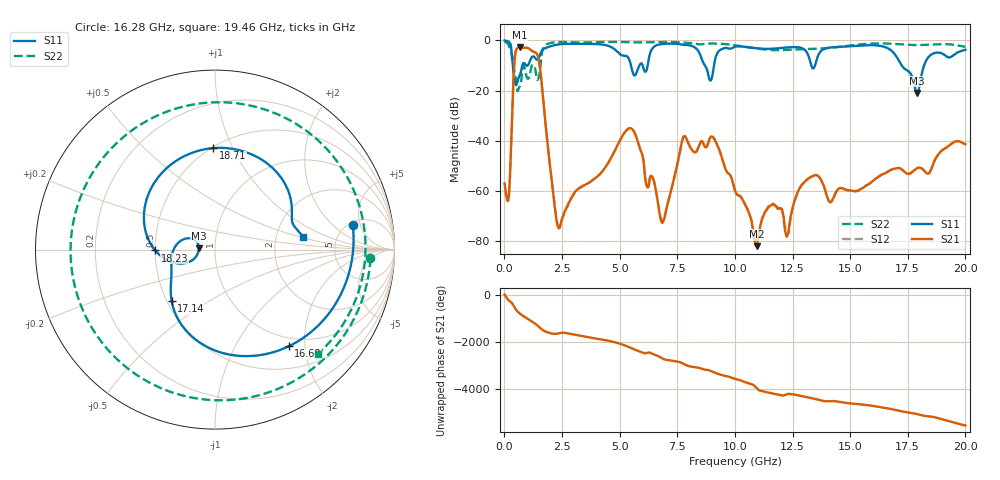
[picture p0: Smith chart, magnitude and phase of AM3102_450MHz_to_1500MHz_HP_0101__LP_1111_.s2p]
!Agilent Technologies,E8364B,MY43040894,A.07.50.67
!Agilent E8364B: A.07.50.67
!Date: Thursday, January 11, 2018 05:43:50
!Correction: S11(Full 2 Port(1,2))
!S21(Full 2 Port(1,2))
!S12(Full 2 Port(1,2))
!S22(Full 2 Port(1,2))
!S2P File: Measurements: S11, S21, S12, S22:
# Hz S  dB  R 50
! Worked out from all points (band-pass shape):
!   1601 points, 10 MHz to 20 GHz, reference 50 ohm
!   highest |S21| = -2.75 dB at 672.2 MHz (marker M1); lowest = -81.9 dB at 10.94 GHz (marker M2)
!   |S21| within 3 dB of the highest: 467 MHz to 1.429 GHz (962 MHz wide, 101 % of centre)
!   lowest |S11| = -20.9 dB at 17.9 GHz (marker M3), VSWR 1.20, Z = 41.7 + j0.587 ohm
!   |S11| at or under -10 dB: 366.7 MHz to 778.1 MHz (411.4 MHz wide, 71.9 % of centre); 8.698 GHz to 9.093 GHz (394.8 MHz wide, 4.44 % of centre); 17.24 GHz to 18.21 GHz (969.7 MHz wide, 5.47 % of centre)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
!   |S22| runs from -20.3 to -0.5 dB; largest |S21 - S12| = 0.0018
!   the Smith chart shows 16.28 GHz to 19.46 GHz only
!   S11 on the Smith chart (normalised r, x): 16.28 GHz: 5.39, +3.77; 16.68 GHz: 0.85, -1.69; 17.14 GHz: 0.53, -0.35; 18.23 GHz: 0.50, -0.01; 18.71 GHz: 0.51, +0.84; 19.46 GHz: 2.87, +0.52
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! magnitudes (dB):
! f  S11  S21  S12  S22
! 10 MHz  -0.1  -56.9  -60.5  -0.5
! 184.9 MHz  -0.6  -62.8  -62.4  -2.0
! 447.3 MHz  -15.9  -7.4  -7.4  -12.9
! 672.2 MHz  -13.8  -2.7  -2.8  -18.2
! 1.484 GHz  -7.1  -7.5  -7.5  -14.9
! 2.334 GHz  -1.7  -74.4  -73.4  -0.7
! 3.346 GHz  -1.4  -58.3  -58.0  -0.9
! 5.47 GHz  -9.2  -34.9  -34.9  -0.8
! 6.682 GHz  -1.7  -66.0  -65.7  -0.7
! 7.819 GHz  -1.8  -38.1  -38.1  -0.9
! 8.931 GHz  -16.0  -38.7  -38.6  -1.3
! 10.01 GHz  -2.5  -59.7  -59.9  -2.0
! 10.94 GHz  -3.2  -81.9  -80.6  -3.2
! 13.34 GHz  -10.6  -54.2  -54.2  -3.4
! 16.28 GHz  -2.2  -53.9  -54.1  -1.2
! 16.68 GHz  -3.4  -52.0  -52.2  -1.3
! 17.14 GHz  -8.5  -50.8  -50.9  -1.6
! 17.9 GHz  -20.9  -50.9  -50.9  -1.9
! 18.23 GHz  -9.5  -52.0  -51.9  -1.8
! 18.71 GHz  -5.0  -46.9  -47.0  -1.6
! 19.46 GHz  -6.1  -40.7  -40.7  -1.8
! 20 GHz  -3.8  -41.3  -41.3  -2.5
